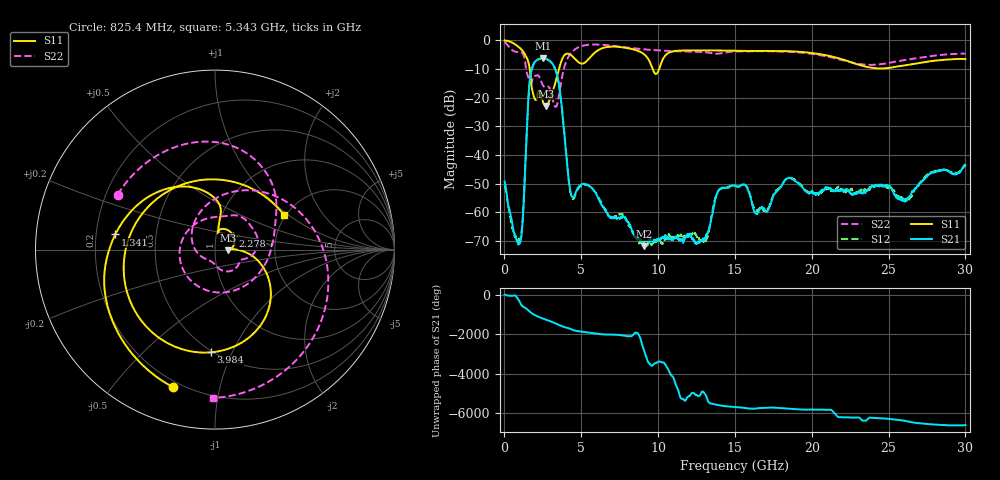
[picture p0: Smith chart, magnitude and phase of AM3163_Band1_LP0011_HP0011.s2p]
!Agilent Technologies,E8364B,MY43040894,A.07.50.67
!Agilent E8364B: A.07.50.67
!Date: Thursday, August 20, 2020 11:17:14
!Correction: S11(Full 2 Port(1,2))
!S21(Full 2 Port(1,2))
!S12(Full 2 Port(1,2))
!S22(Full 2 Port(1,2))
!S2P File: Measurements: S11, S21, S12, S22:
# Hz S  dB  R 50
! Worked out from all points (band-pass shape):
!   3201 points, 10 MHz to 30 GHz, reference 50 ohm
!   highest |S21| = -6.27 dB at 2.503 GHz (marker M1); lowest = -71.9 dB at 9.073 GHz (marker M2)
!   |S21| within 3 dB of the highest: 1.832 GHz to 3.239 GHz (1.407 GHz wide, 55.5 % of centre)
!   lowest |S11| = -23.0 dB at 2.69 GHz (marker M3), VSWR 1.15, Z = 57.6 - j0.374 ohm
!   |S11| at or under -10 dB: 1.647 GHz to 3.554 GHz (1.907 GHz wide, 73.3 % of centre); 9.643 GHz to 10.07 GHz (427.8 MHz wide, 4.34 % of centre)
!   |S22| runs from -23.3 to -0.6 dB; largest |S21 - S12| = 0.0049
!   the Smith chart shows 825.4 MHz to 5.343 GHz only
!   S11 on the Smith chart (normalised r, x): 825.4 MHz: 0.17, -0.73; 1.341 GHz: 0.28, +0.07; 2.278 GHz: 1.21, +0.19; 3.984 GHz: 0.49, -0.83; 5.343 GHz: 1.97, +0.92
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1e7  -0.07 -8.5  -49.29 -0.7  -50.69 -47.4  -0.57 -26.3
8.253531e8  -1.93 -107.0  -69.98 -166.6  -69.35 -162.9  -4.12 150.6
1.340806e9  -5.00 171.4  -45.75 52.4  -45.73 46.1  -7.25 38.1
1.696938e9  -12.68 82.1  -12.33 -178.3  -12.33 -178.4  -14.77 137.5
2.277994e9  -17.90 37.2  -6.49 -65.7  -6.49 -65.7  -12.89 -1.6
2.502919e9  -21.50 -0.5  -6.27 -133.7  -6.27 -133.7  -15.69 -19.3
2.690356e9  -22.97 -2.6  -6.46 172.4  -6.47 172.4  -16.35 -26.1
3.449478e9  -12.07 -14.8  -12.73 -63.9  -12.75 -63.8  -22.04 -144.8
3.983675e9  -4.83 -92.5  -37.80 140.7  -37.70 139.8  -7.88 54.0
4.386666e9  -5.43 -159.7  -54.51 28.9  -55.03 28.6  -4.14 -5.3
5.014581e9  -8.16 87.8  -50.24 -79.4  -50.69 -79.3  -2.04 -65.9
5.342597e9  -7.32 26.2  -50.30 -114.2  -50.51 -114.1  -1.65 -90.6
6.439106e9  -2.65 -103.3  -58.34 146.5  -58.01 147.1  -1.61 -155.5
7.554359e9  -2.38 -177.3  -61.71 107.3  -60.66 104.9  -2.25 153.7
9.072603e9  -4.82 101.8  -71.86 89.7  -70.53 -30.3  -3.15 93.8
1.000979e10  -10.82 109.1  -69.75 -147.4  -69.65 -147.3  -3.55 59.2
1.239025e10  -3.54 7.8  -70.61 5.0  -67.42 -87.0  -3.98 -22.2
1.5005e10  -3.65 -72.1  -50.74 66.1  -50.85 68.0  -3.92 -90.3
2.000958e10  -4.43 163.3  -52.92 -55.2  -52.89 -61.8  -4.71 136.7
2.275554e10  -8.04 60.2  -53.54 -104.6  -53.02 -97.4  -7.98 21.2
2.500479e10  -9.67 -62.2  -50.83 -164.7  -51.68 -167.2  -7.96 -92.1
3e10  -6.60 104.2  -43.68 -121.8  -43.20 -133.0  -4.65 102.4
